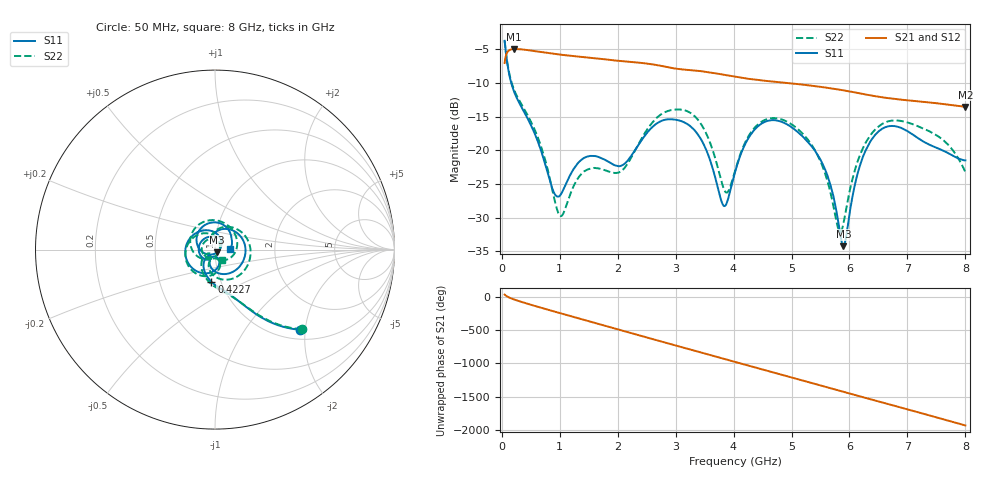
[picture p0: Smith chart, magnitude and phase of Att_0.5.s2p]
#  HZ  S  DB  R  50.00
! Rohde & Schwarz Vector Network Analyzer
! Rohde-Schwarz,ZNB40-4Port,1311601084101679,3.45
! Created: UTC 4/25/2025, 9:28:04 AM
! freq[Hz]  db:S11  ang:S11  db:S21  ang:S21  db:S12  ang:S12  db:S22  ang:S22
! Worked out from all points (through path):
!   1750 points, 50 MHz to 8 GHz, reference 50 ohm
!   highest |S21| = -4.93 dB at 213.6 MHz (marker M1); lowest = -13.5 dB at 8 GHz (marker M2)
!   group delay of S21, straight-line fit = 669 ps
!   lowest |S11| = -34.2 dB at 5.895 GHz (marker M3), VSWR 1.04, Z = 51.2 - j1.59 ohm
!   |S11| at or under -10 dB: 165.2 MHz to end of sweep
!   |S22| runs from -32.2 to -3.7 dB; largest |S21 - S12| = 0.00066
!   S11 on the Smith chart (normalised r, x): 50 MHz: 1.21, -1.88; 422.7 MHz: 0.90, -0.34; 8 GHz: 1.18, +0.01
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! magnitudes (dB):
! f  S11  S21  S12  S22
! 50 MHz  -3.7  -7.0  -7.0  -3.7
! 213.6 MHz  -11.3  -4.9  -4.9  -11.0
! 422.7 MHz  -14.9  -5.1  -5.1  -14.4
! 681.8 MHz  -20.1  -5.4  -5.4  -19.5
! 890.9 MHz  -26.1  -5.6  -5.6  -26.5
! 1 GHz  -26.8  -5.8  -5.8  -29.7
! 1.377 GHz  -21.4  -6.1  -6.1  -23.5
! 2.064 GHz  -22.3  -6.7  -6.7  -23.1
! 2.7 GHz  -15.9  -7.4  -7.4  -15.0
! 3.359 GHz  -17.3  -8.2  -8.2  -15.2
! 3.832 GHz  -28.2  -8.8  -8.8  -25.7
! 4.027 GHz  -23.2  -9.1  -9.1  -23.0
! 4.273 GHz  -18.0  -9.4  -9.4  -17.7
! 4.577 GHz  -15.6  -9.7  -9.7  -15.4
! 5.35 GHz  -19.4  -10.4  -10.4  -19.2
! 5.636 GHz  -24.1  -10.7  -10.7  -25.1
! 5.809 GHz  -30.7  -10.9  -10.9  -31.7
! 5.895 GHz  -34.2  -11.1  -11.1  -30.9
! 6.236 GHz  -20.9  -11.6  -11.6  -19.6
! 6.677 GHz  -16.4  -12.2  -12.2  -15.7
! 7.518 GHz  -19.7  -13.0  -13.0  -17.8
! 8 GHz  -21.5  -13.5  -13.5  -23.2
